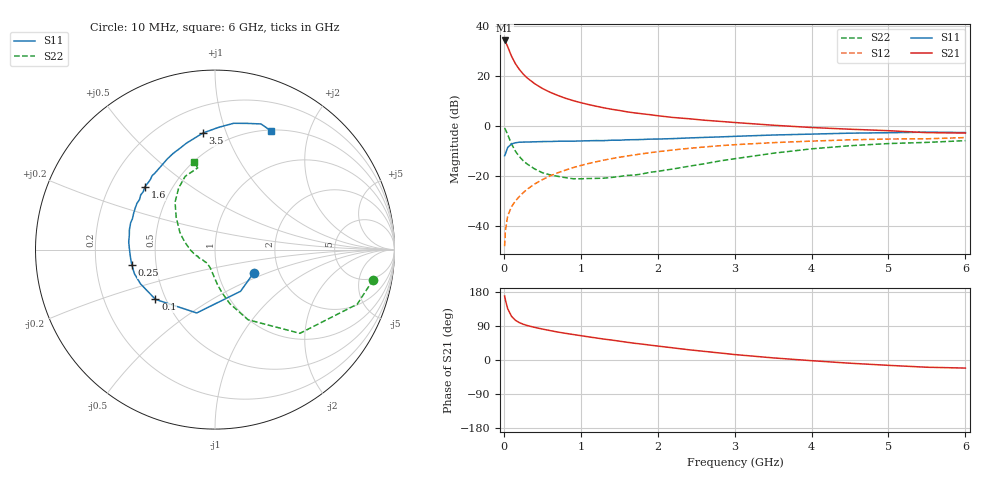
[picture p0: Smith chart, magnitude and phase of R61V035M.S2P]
! SIEMENS Small Signal Semiconductors
! BFR193
! Si NPN RF Bipolar Junction Transistor in SOT23
! VCE = 1 V  IC = 35 mA
! Common Emitter S-Parameters:  May  1996
# GHz  S  MA  R  50
!  f  S11  S21  S12  S22
! GHz  MAG  ANG  MAG  ANG  MAG  ANG  MAG  ANG
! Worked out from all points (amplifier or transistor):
!   36 points, 10 MHz to 6 GHz, reference 50 ohm
!   highest |S21| = 34.1 dB at 10 MHz (marker M1)
!   |S21| within 3 dB of that: start of sweep to 56.53 MHz
!   unconditionally stable (mu >= 1): 353.4 MHz to 2.223 GHz
!   at 250 MHz: K = 0.95, MSG = 23.8 dB, |S12| = -26.8 dB
!   at 1.4 GHz: K = 1.03, MAG = 8.8 dB, |S12| = -13.2 dB
!   at 6 GHz: K = 0.98, MSG = 0.9 dB, |S12| = -4.7 dB
!   S11 on the Smith chart (normalised r, x): 10 MHz: 1.48, -0.41; 100 MHz: 0.44, -0.30; 250 MHz: 0.36, -0.08; 1.6 GHz: 0.35, +0.34; 3.5 GHz: 0.37, +0.83; 6 GHz: 0.51, +1.45
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0.01  0.2516 -31.4  50.92 169.0  0.0039 81.7  0.8974 -10.7
0.02  0.2724 -58.5  48.67 158.6  0.0079 76.9  0.8487 -21.0
0.05  0.3675 -106.1  38.17 135.3  0.0157 66.8  0.6644 -44.6
0.1  0.4323 -140.1  24.61 115.3  0.0241 64.0  0.4319 -64.8
0.15  0.4567 -155.3  17.51 104.9  0.0311 64.7  0.3106 -74.8
0.2  0.4687 -163.4  13.51 98.8  0.0382 67.5  0.2434 -80.7
0.25  0.4712 -169.4  10.9 94.5  0.0456 69.3  0.2007 -85.4
0.3  0.4728 -173.9  9.152 91.2  0.0532 69.9  0.1731 -88.6
0.4  0.4773 179.2  6.957 86.1  0.0683 71.2  0.137 -94.8
0.5  0.4826 174.9  5.596 81.7  0.0833 71.2  0.1152 -100.6
0.6  0.4842 170.4  4.69 77.7  0.0992 70.6  0.1042 -105.1
0.7  0.4898 166.7  4.053 73.8  0.1144 70.1  0.0974 -110.1
0.8  0.493 162.5  3.557 70.5  0.1297 68.6  0.0916 -115.9
1.1  0.5009 152.7  2.661 61.1  0.1757 65.0  0.088 -129.9
1.3  0.5045 146.5  2.287 55.2  0.2054 62.0  0.0894 -140.1
1.6  0.5245 138.2  1.902 46.9  0.2482 57.3  0.1015 -154.1
2.2  0.5536 122.9  1.466 32.0  0.3283 47.6  0.1367 -178.9
3  0.6142 105.0  1.163 14.4  0.4183 34.1  0.2192 153.5
3.5  0.653 95.9  1.026 5.6  0.4596 26.0  0.282 140.1
4.5  0.7114 81.6  0.853 -8.5  0.5227 11.9  0.3987 120.5
5.5  0.7455 69.9  0.728 -19.1  0.5488 -1.5  0.4651 102.0
6  0.7314 64.8  0.716 -21.3  0.5803 -5.5  0.5037 103.4
